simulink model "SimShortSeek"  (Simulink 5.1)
settings: Solver=ode45  StartTime=0.0  StopTime=NmaxTs*Ts  RelTol=1e-3
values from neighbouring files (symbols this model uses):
  FlutterDist = SetFlutterDist(PlantData,DistParam)    [HDDBench.m]
  ForceDist = SetForceDist(PlantData,DistParam)    [HDDBench.m]
  g_flutter = 1    [example3.m]    (also in followdemo.m)
  g_rro = 1    [example3.m]    (also in followdemo.m)
  g_sensor = 1    [example3.m]    (also in followdemo.m)
  g_torque = 1    [example3.m]    (also in followdemo.m)
  RRO = SetRRO(PlantData,DistParam)    [HDDBench.m]
  SeekLength = 100    [example3.m]
  SensorNoise = SetSensorNoise(PlantData,DistParam)    [HDDBench.m]
  sys_dP = c2d(sys_P, Tsn)    [example3.m]
  Tc = Ts/2    [example3.m]    (also in hdd_plantparam.m = 3.78787878788e-05; followdemo.m)
  Ts = PlantData.Ts    [example3.m]    (also in HDDBenchPlot.m; hdd_plantparam.m = 3.78787878788e-05; SetDistParam.m; SetFlutterDist.m)

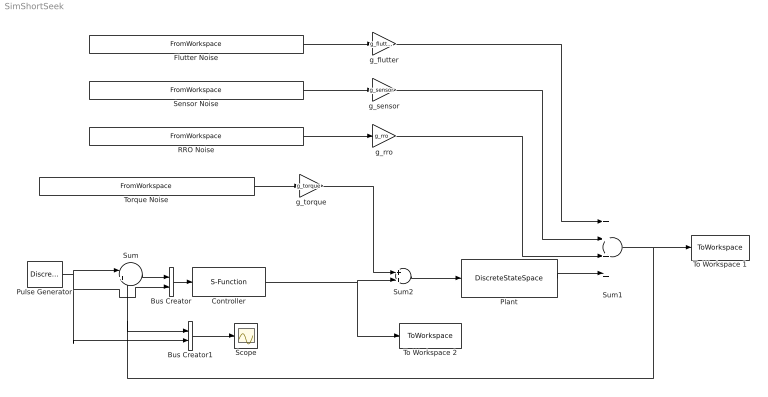
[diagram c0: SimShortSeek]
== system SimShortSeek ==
  Bus Creator : BusCreator  Inputs=2
  Bus Creator1 : BusCreator  Inputs=2
  Controller : S-Function  FunctionName=Controller  Parameters=CtrlPar
  Flutter Noise : FromWorkspace  VariableName=[FlutterDist.Time, FlutterDist.Data]  SampleTime=FlutterDist.Ts  Interpolate=off  OutputAfterFinalValue=Setting to zero
  Plant : DiscreteStateSpace  A=sys_dP.a  B=sys_dP.b  C=sys_dP.c  D=sys_dP.d  SampleTime=sys_dP.Ts
  Pulse Generator : DiscretePulseGenerator  PulseType=Time based  Amplitude=SeekLength  Period=0.1  PulseWidth=50  SampleTime=Ts
  RRO Noise : FromWorkspace  VariableName=[RRO.Time,RRO.Data]  SampleTime=RRO.Ts  Interpolate=off  OutputAfterFinalValue=Setting to zero
  Scope : Scope
  Sensor Noise : FromWorkspace  VariableName=[SensorNoise.Time,SensorNoise.Data]  SampleTime=SensorNoise.Ts  Interpolate=off  OutputAfterFinalValue=Setting to zero
  Sum : Sum  Inputs=|+-  ShowAdditionalParam=on
  Sum1 : Sum  Inputs=+++|+
  Sum2 : Sum  ShowAdditionalParam=on
  To Workspace 1 : ToWorkspace  VariableName=PESDataT  SampleTime=Ts  SaveFormat=StructureWithTime
  To Workspace 2 : ToWorkspace  VariableName=ControlDataT  SampleTime=Tc  SaveFormat=StructureWithTime
  Torque Noise : FromWorkspace  VariableName=[ForceDist.Time, ForceDist.Data]  SampleTime=ForceDist.Ts  Interpolate=off  OutputAfterFinalValue=Setting to zero
  g_flutter : Gain  Gain=g_flutter
  g_rro : Gain  Gain=g_rro
  g_sensor : Gain  Gain=g_sensor
  g_torque : Gain  Gain=g_torque
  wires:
  Pulse Generator/1 -> Sum/1, Bus Creator/2, Bus Creator1/2
  Controller/1 -> Sum2/2, To Workspace 2/1
  Sum1/1 -> To Workspace 1/1, Sum/2, Bus Creator1/1
  g_torque/1 -> Sum2/1
  Torque Noise/1 -> g_torque/1
  Sensor Noise/1 -> g_sensor/1
  g_sensor/1 -> Sum1/2
  Flutter Noise/1 -> g_flutter/1
  g_flutter/1 -> Sum1/1
  RRO Noise/1 -> g_rro/1
  g_rro/1 -> Sum1/3
  Plant/1 -> Sum1/4
  Sum2/1 -> Plant/1
  Bus Creator/1 -> Controller/1
  Sum/1 -> Bus Creator/1
  Bus Creator1/1 -> Scope/1
